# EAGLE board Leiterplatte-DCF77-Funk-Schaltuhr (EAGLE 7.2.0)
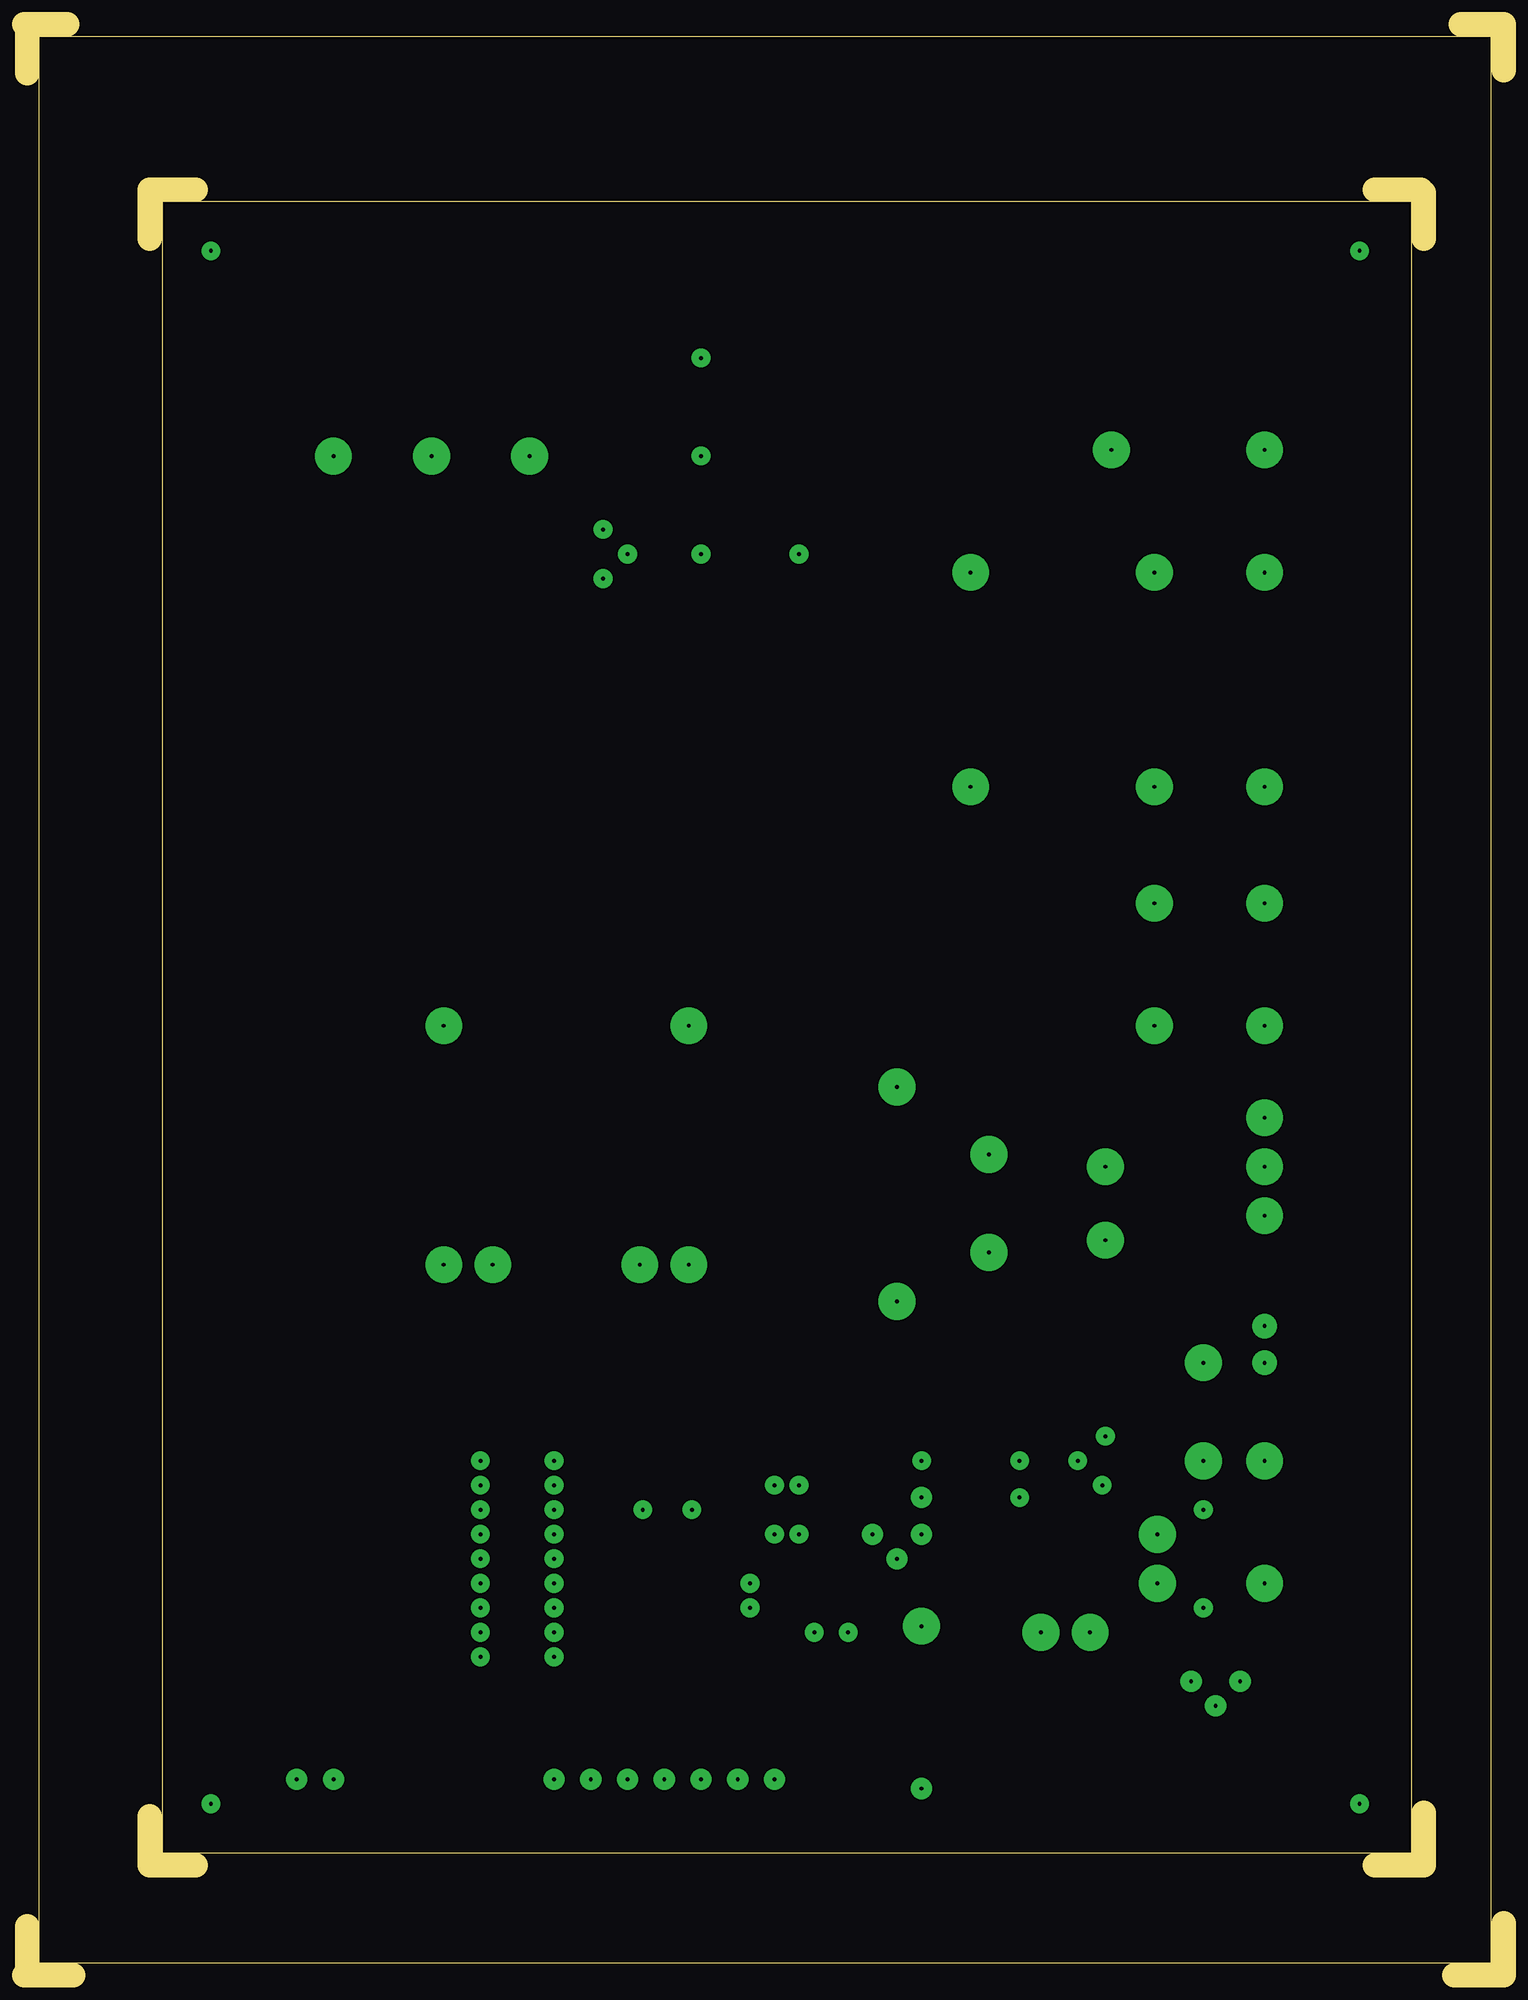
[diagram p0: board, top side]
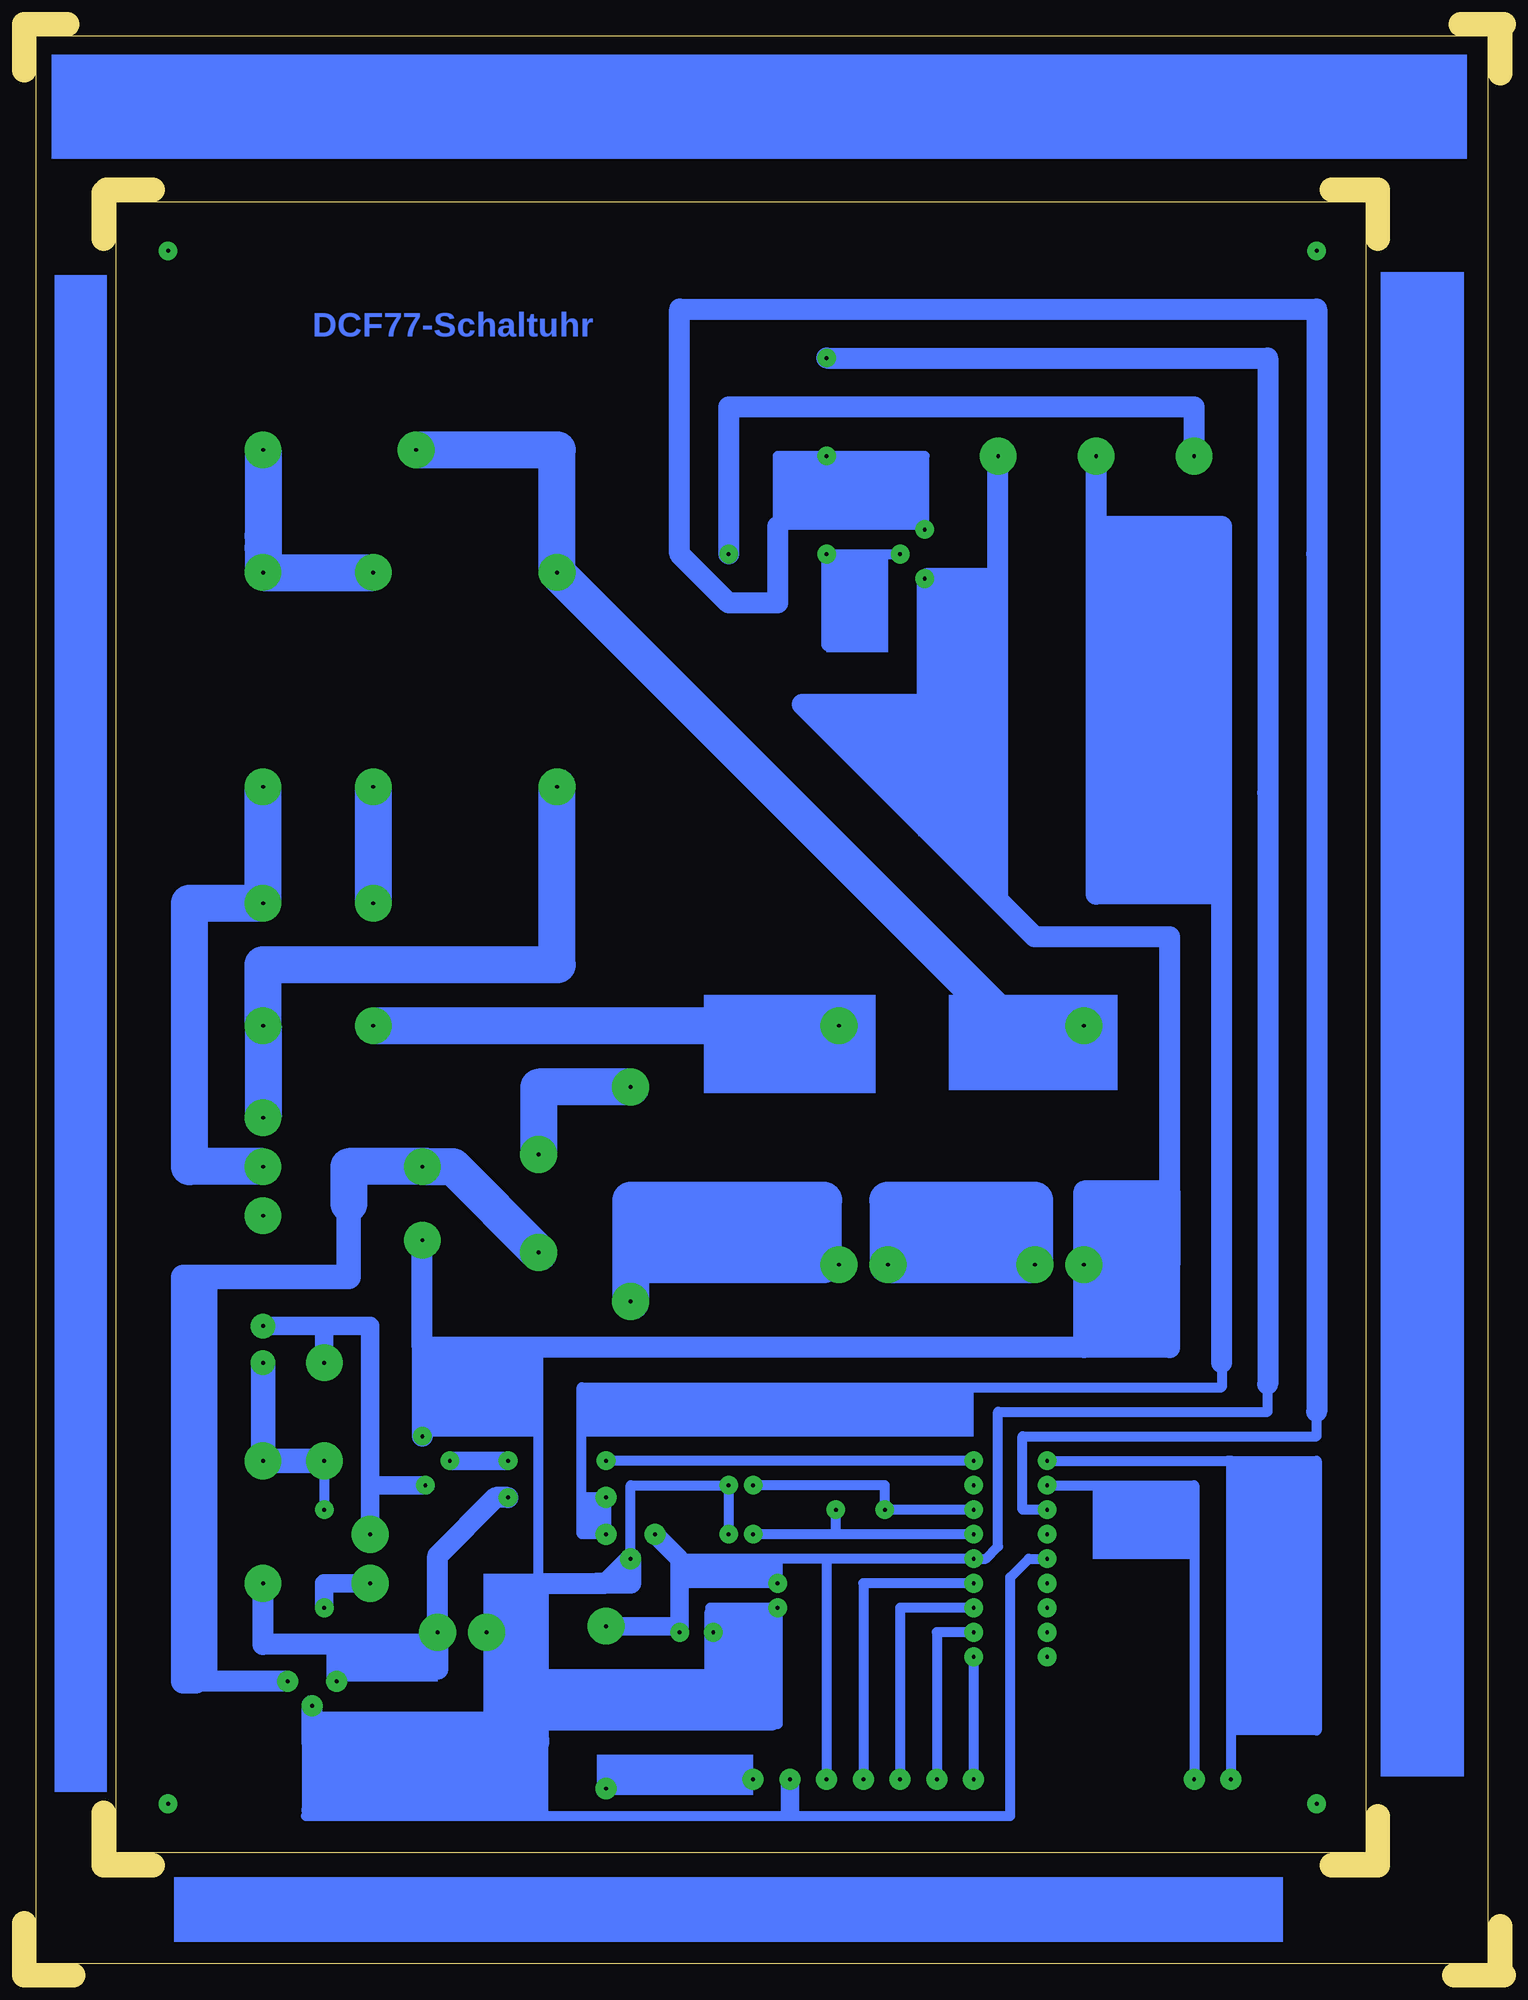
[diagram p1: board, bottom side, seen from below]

Size 153.35 x 202.25 mm. Coordinates in mm from the lower left corner, seen from the top.
Outline: 153.35,5.4 153.35,0.32
Outline: 153.35,0 148.27,0
Outline: 153.35,197.49 153.35,202.25 148.91,202.25
Outline: 0.32,5.08 0.32,0
Outline: 5.08,0 0.32,0
Outline: 0.32,0 0,0
Outline: 4.44,202.25 0,202.25
Outline: 0.32,197.17 0.32,201.93
Outline: 17.78,11.43 13.02,11.43
Outline: 13.02,16.51 13.02,11.75
Outline: 145.1,11.43 140.02,11.43
Outline: 145.1,16.83 145.1,11.75
Outline: 145.1,180.02 145.1,184.78
Outline: 144.78,185.1 140.02,185.1
Outline: 13.02,180.02 13.02,184.78
Outline: 17.78,185.1 13.02,185.1
Outline: 152.08,1.27 152.08,200.98 1.59,200.98 1.59,1.27 152.08,1.27
Outline: 14.29,12.7 143.83,12.7 143.83,183.83 14.29,183.83 14.29,12.7
Copper layers (1*16): Top 0.035mm / dielectric 1.5mm / Bottom 0.035mm
Design rules "default": minimum track width 10mil, minimum drill 24mil, track to track 8mil, track to pad 8mil, pad to pad 8mil, via to via 8mil, smd to smd 8mil, copper to edge 40mil, drill to drill 8mil, minimum pad ring 10mil, minimum via ring 8mil, stop-mask expansion 4mil, vias tented up to drill 0mil, thermal gap 10mil

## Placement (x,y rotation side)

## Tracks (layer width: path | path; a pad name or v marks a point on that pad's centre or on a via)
S$2  (via drill 0.4 pad 1.93)
  other vias: 19.37,17.78
S$4  (via drill 0.4 pad 1.93)
  other vias: 19.37,178.75
S$5  (via drill 0.4 pad 1.93)
  other vias: 138.43,178.75
S$6  (via drill 0.4 pad 1.93)
  other vias: 138.43,17.78
S$7  (via drill 0.4 pad 3.81)
  Bottom 3.81: v48.58,73.66 v63.82,73.66 63.82,80.33 48.58,80.33 v48.58,73.66
S$8  (via drill 0.4 pad 3.81)
  Bottom 3.81: 90.49,73.34 90.49,73.66 70.48,73.66 70.48,80.33 90.49,80.33 90.49,73.34 | 90.49,73.34 v90.49,69.85
S$9  (via drill 0.4 pad 3.81)
  Bottom 3.81: v117.16,123.19 v117.16,111.12
S$10  (via drill 0.4 pad 3.81)
  other vias: 117.16,98.42
S$11  (via drill 0.4 pad 3.81)
  Bottom 3.81: v68.9,98.42 116.52,98.42
S$12  (via drill 0.4 pad 1.93, 0.4 pad 3.81)
  Bottom 2.184: v32.07,157.48 32.07,162.56 80.33,162.56 v80.33,147.32
S$13  (via drill 0.4 pad 3.81)
  Bottom 3.81: v98.11,123.19 98.11,104.77 128.59,104.77 v128.59,98.42 v128.59,88.9
S$14  (via drill 0.4 pad 1.93)
  other vias: 85.41,35.56
S$15  (via drill 0.4 pad 3.81)
  Bottom 3.81: v128.59,158.12 128.59,149.23 | 128.59,149.23 128.59,147.96 | v117.16,145.42 v128.59,145.42 128.59,149.23
S$16  (via drill 0.4 pad 1.93)
  Bottom 1.016: v47.31,53.34 28.58,53.34 | 28.58,53.34 28.26,53.34 28.26,25.4 | 28.26,25.4 28.26,20.32 | 28.58,53.34 19.37,53.34 19.37,25.4 28.26,25.4
S$17  (via drill 0.4 pad 1.93, 0.4 pad 2.18)
  Bottom 1.016: v47.31,50.8 32.07,50.8 v32.07,20.32
S$18  (via drill 0.4 pad 3.81)
  Bottom 3.81: v112.71,158.12 98.11,158.12 v98.11,145.42 51.12,98.42 v43.5,98.42
S$19  (via drill 0.4 pad 1.93, 0.4 pad 2.18, 0.4 pad 3.81)
  Bottom 2.184: v128.59,40.64 128.59,34.29 120.97,34.29 | v110.49,35.56 110.49,43.5 104.46,49.53 v103.19,49.53 | 120.97,34.29 v120.97,30.48 | 120.97,34.29 110.49,34.29 v110.49,35.56 | v110.49,35.56 110.49,31.75
S$20  (via drill 0.4 pad 1.93)
  other vias: 47.31,45.72
S$21  (via drill 0.4 pad 1.93)
  Bottom 1.016: v47.31,43.18 49.21,43.18 51.12,41.28 51.12,23.81
S$22  (via drill 0.4 pad 1.93)
  other vias: 47.31,40.64
S$23  (via drill 0.4 pad 2.18)
  Bottom 1.016: v77.79,20.32 92.07,20.32 v93.03,19.37
S$24  (via drill 0.4 pad 1.93)
  other vias: 47.31,35.56
S$25  (via drill 0.4 pad 1.93)
  other vias: 47.31,33.02
S$26  (via drill 0.4 pad 1.93)
  Bottom 1.016: v54.93,53.34 v93.03,53.34
S$27  (via drill 0.4 pad 1.93)
  other vias: 54.93,50.8
S$28  (via drill 0.4 pad 1.93)
  Bottom 1.016: v54.93,48.26 v64.13,48.26 64.13,50.8 v77.79,50.8
S$29  (via drill 0.4 pad 1.93)
  Bottom 1.016: v54.93,45.72 69.21,45.72 | 69.21,45.72 v69.21,48.26 | 69.21,45.72 v77.79,45.72
S$30  (via drill 0.4 pad 3.81)
  other vias: 68.9,73.66
S$31  (via drill 0.4 pad 1.93, 0.4 pad 2.18)
  Bottom 1.016: v54.93,40.64 66.36,40.64 v66.36,20.32
S$32  (via drill 0.4 pad 1.93, 0.4 pad 2.18)
  Bottom 1.016: v54.93,38.1 62.55,38.1 v62.55,20.32
S$33  (via drill 0.4 pad 1.93, 0.4 pad 2.18)
  Bottom 1.016: v54.93,35.56 58.74,35.56 v58.74,20.32
S$34  (via drill 0.4 pad 1.93, 0.4 pad 2.18)
  Bottom 1.016: v54.93,33.02 v54.93,20.32
S$35  (via drill 0.4 pad 1.93, 0.4 pad 2.18)
  Bottom 1.016: 75.25,35.88 v75.25,38.1 82.23,38.1 82.23,35.56 | 75.25,35.88 75.25,35.56 v81.92,35.56 | v80.33,45.72 v80.33,50.8 90.49,50.8 v90.49,43.18 | 100.01,40.64 100.01,64.77 | 100.01,24.45 100.01,16.51 99.7,16.51 | 99.7,16.51 51.12,16.51 51.12,23.5 | 99.7,16.51 124.14,16.51 | 75.25,35.88 75.25,26.04 82.23,26.04
  Bottom 1.93: 81.92,31.11 v81.92,35.56 81.92,37.47 | 81.92,31.11 81.92,30.8 99.7,30.8 | 81.92,31.11 81.92,26.35 82.23,26.35 | 100.01,40.64 100.01,35.56 | 82.23,26.35 100.01,26.35 | 82.23,26.35 75.88,26.35
  Bottom 2.184: 123.51,25.4 123.51,24.13 100.01,24.13 100.01,24.45 100.01,26.35 100.01,40.64 93.98,40.64 | 123.51,25.4 v123.51,27.94 | 93.98,40.64 93.03,40.64 v90.49,43.18 90.49,40.64 93.98,40.64 | 123.51,25.4 123.51,17.14
S$36  (via drill 0.4 pad 3.81)
  Bottom 3.81: v90.49,92.08 100.01,92.08 v100.01,85.09
S$37  (via drill 0.4 pad 1.93)
  other vias: 47.31,38.1
S$38  (via drill 0.4 pad 3.81)
  Bottom 2.184: v105.41,35.56 100.33,35.56
S$39  (via drill 0.4 pad 1.93)
  Bottom 1.93: v103.19,53.34 v109.22,53.34
S$40  (via drill 0.4 pad 2.18, 0.4 pad 3.81)
  Bottom 2.184: v126.05,30.48 135.89,30.48
  Bottom 2.54: 119.06,83.82 v112.08,83.82 | 119.7,80.01 119.7,72.39 136.84,72.39 136.84,30.48 135.89,30.48 135.57,30.48
  Bottom 3.81: v100.01,74.93 108.9,83.82 111.44,83.82 | v112.08,83.82 111.44,83.82 | 111.44,83.82 119.06,83.82 119.7,83.82 119.7,80.01
S$42  (via drill 0.4 pad 3.81)
  Bottom 3.81: v128.59,83.82 136.21,83.82 136.21,111.12 v128.59,111.12 v128.59,123.19
S$43  (via drill 0.4 pad 3.81)
  other vias: 128.59,78.74
S$47  (via drill 0.4 pad 1.93, 0.4 pad 2.54, 0.4 pad 3.81)
  Bottom 1.016: v122.24,53.34 v122.24,48.26
  Bottom 2.54: v128.59,63.5 v128.59,53.34 v122.24,53.34
S$48  (via drill 0.4 pad 2.18)
  Bottom 1.016: 95.57,49.85 95.57,49.53 v93.03,49.53 v93.03,45.72 95.57,45.72 95.57,49.85 | 95.57,49.85 95.57,60.96 29.21,60.96
S$49  (via drill 0.4 pad 1.93, 0.4 pad 2.54, 0.4 pad 3.81)
  Bottom 1.93: v128.59,67.31 122.24,67.31 | 122.24,67.31 117.48,67.31 117.48,50.8 | 117.48,50.8 v111.76,50.8 | 122.24,67.31 v122.24,63.5 | v117.48,45.72 117.48,50.8
S$50  (via drill 0.4 pad 1.93, 0.4 pad 3.81)
  Bottom 1.93: v117.48,40.64 122.24,40.64 v122.24,38.1
S$52  (via drill 0.4 pad 2.18, 0.4 pad 3.81)
  Bottom 1.93: v87.95,45.72 85.41,43.18 85.41,36.2 v93.03,36.2
S$53  (via drill 0.4 pad 3.81)
  other vias: 52.39,157.48
S$55  (via drill 0.4 pad 3.81)
  Bottom 1.016: 29.21,63.5 29.21,60.96
  Bottom 2.184: 29.21,63.5 29.21,111.76 | 29.21,111.76 29.21,112.08 42.23,112.08 42.23,150.18 | 42.23,150.18 v42.23,157.48 | 29.21,111.76 29.21,150.18 42.23,150.18
S$56  (via drill 0.4 pad 2.18)
  other vias: 28.26,20.32
S$57  (via drill 0.4 pad 2.18)
  Bottom 1.016: 73.98,17.14 73.98,16.83
  Bottom 1.93: v73.98,20.32 73.98,17.14
S$59  (via drill 0.4 pad 1.93, 0.4 pad 3.81)
  Bottom 1.016: 34.61,89.53 34.61,94.61 | 34.61,89.53 34.61,89.22 | 34.61,82.55 34.61,89.53 | v43.5,73.66 43.5,73.98 | 52.7,157.48 52.39,157.48 52.39,144.78 | 52.39,144.78 52.39,137.16 | 52.39,137.16 52.39,111.76 | 52.39,137.16 60.01,137.16 | 52.39,144.78 53.02,144.78 | 59.69,144.78 v60.01,144.78
  Bottom 2.184: 112.08,65.09 v112.08,76.2 | 43.5,65.41 v43.5,73.66 | 43.5,65.09 112.08,65.09 | 112.08,65.09 v112.08,55.88 | v43.5,73.66 34.61,73.66 34.61,81.28 | 34.61,81.28 34.61,82.55 34.61,94.61 34.61,107.63 48.58,107.63 52.39,111.44 | 52.39,111.44 52.39,157.48 | 52.39,111.44 72.71,131.76 59.69,131.76 59.69,144.78 53.02,144.78 | v43.5,73.66 43.5,81.28 34.61,81.28 | 34.61,81.28 34.61,65.41 43.5,65.41 | 43.5,65.09 43.5,65.41 | 34.61,65.09 43.5,65.09
S$60  (via drill 0.4 pad 1.93)
  Bottom 1.016: v60.01,149.86 60.01,157.48 v70.17,157.48 75.25,157.48 75.25,150.18 | v47.31,48.26 49.85,48.26 49.85,55.88 19.37,55.88 19.37,58.42
  Bottom 2.184: 75.25,150.18 75.25,142.24 80.33,142.24 85.41,147.32 85.41,172.72 19.37,172.72 19.37,147.32 19.37,58.42
S$62  (via drill 0.4 pad 1.93)
  Bottom 1.016: v62.55,147.32 v70.17,147.32 70.17,137.8
S$68  (via drill 0.4 pad 1.93, 0.4 pad 2.18)
  Bottom 1.016: 70.17,43.18 v54.93,43.18 53.66,43.18 52.39,44.45 52.39,58.42 24.45,58.42 24.45,61.28 | 70.17,43.18 75.25,43.18 | 75.25,43.18 85.09,43.18 | 75.25,43.18 v75.25,40.64 85.09,40.64 | 70.17,43.18 v70.17,20.32 | v70.17,167.64 70.48,167.64
  Bottom 2.184: v70.17,167.64 24.45,167.64 24.45,122.55 24.45,61.28
(copper drawn outside any net)
  shapes: Bottom area x43

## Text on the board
Bottom: DCF77-Schaltuhr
